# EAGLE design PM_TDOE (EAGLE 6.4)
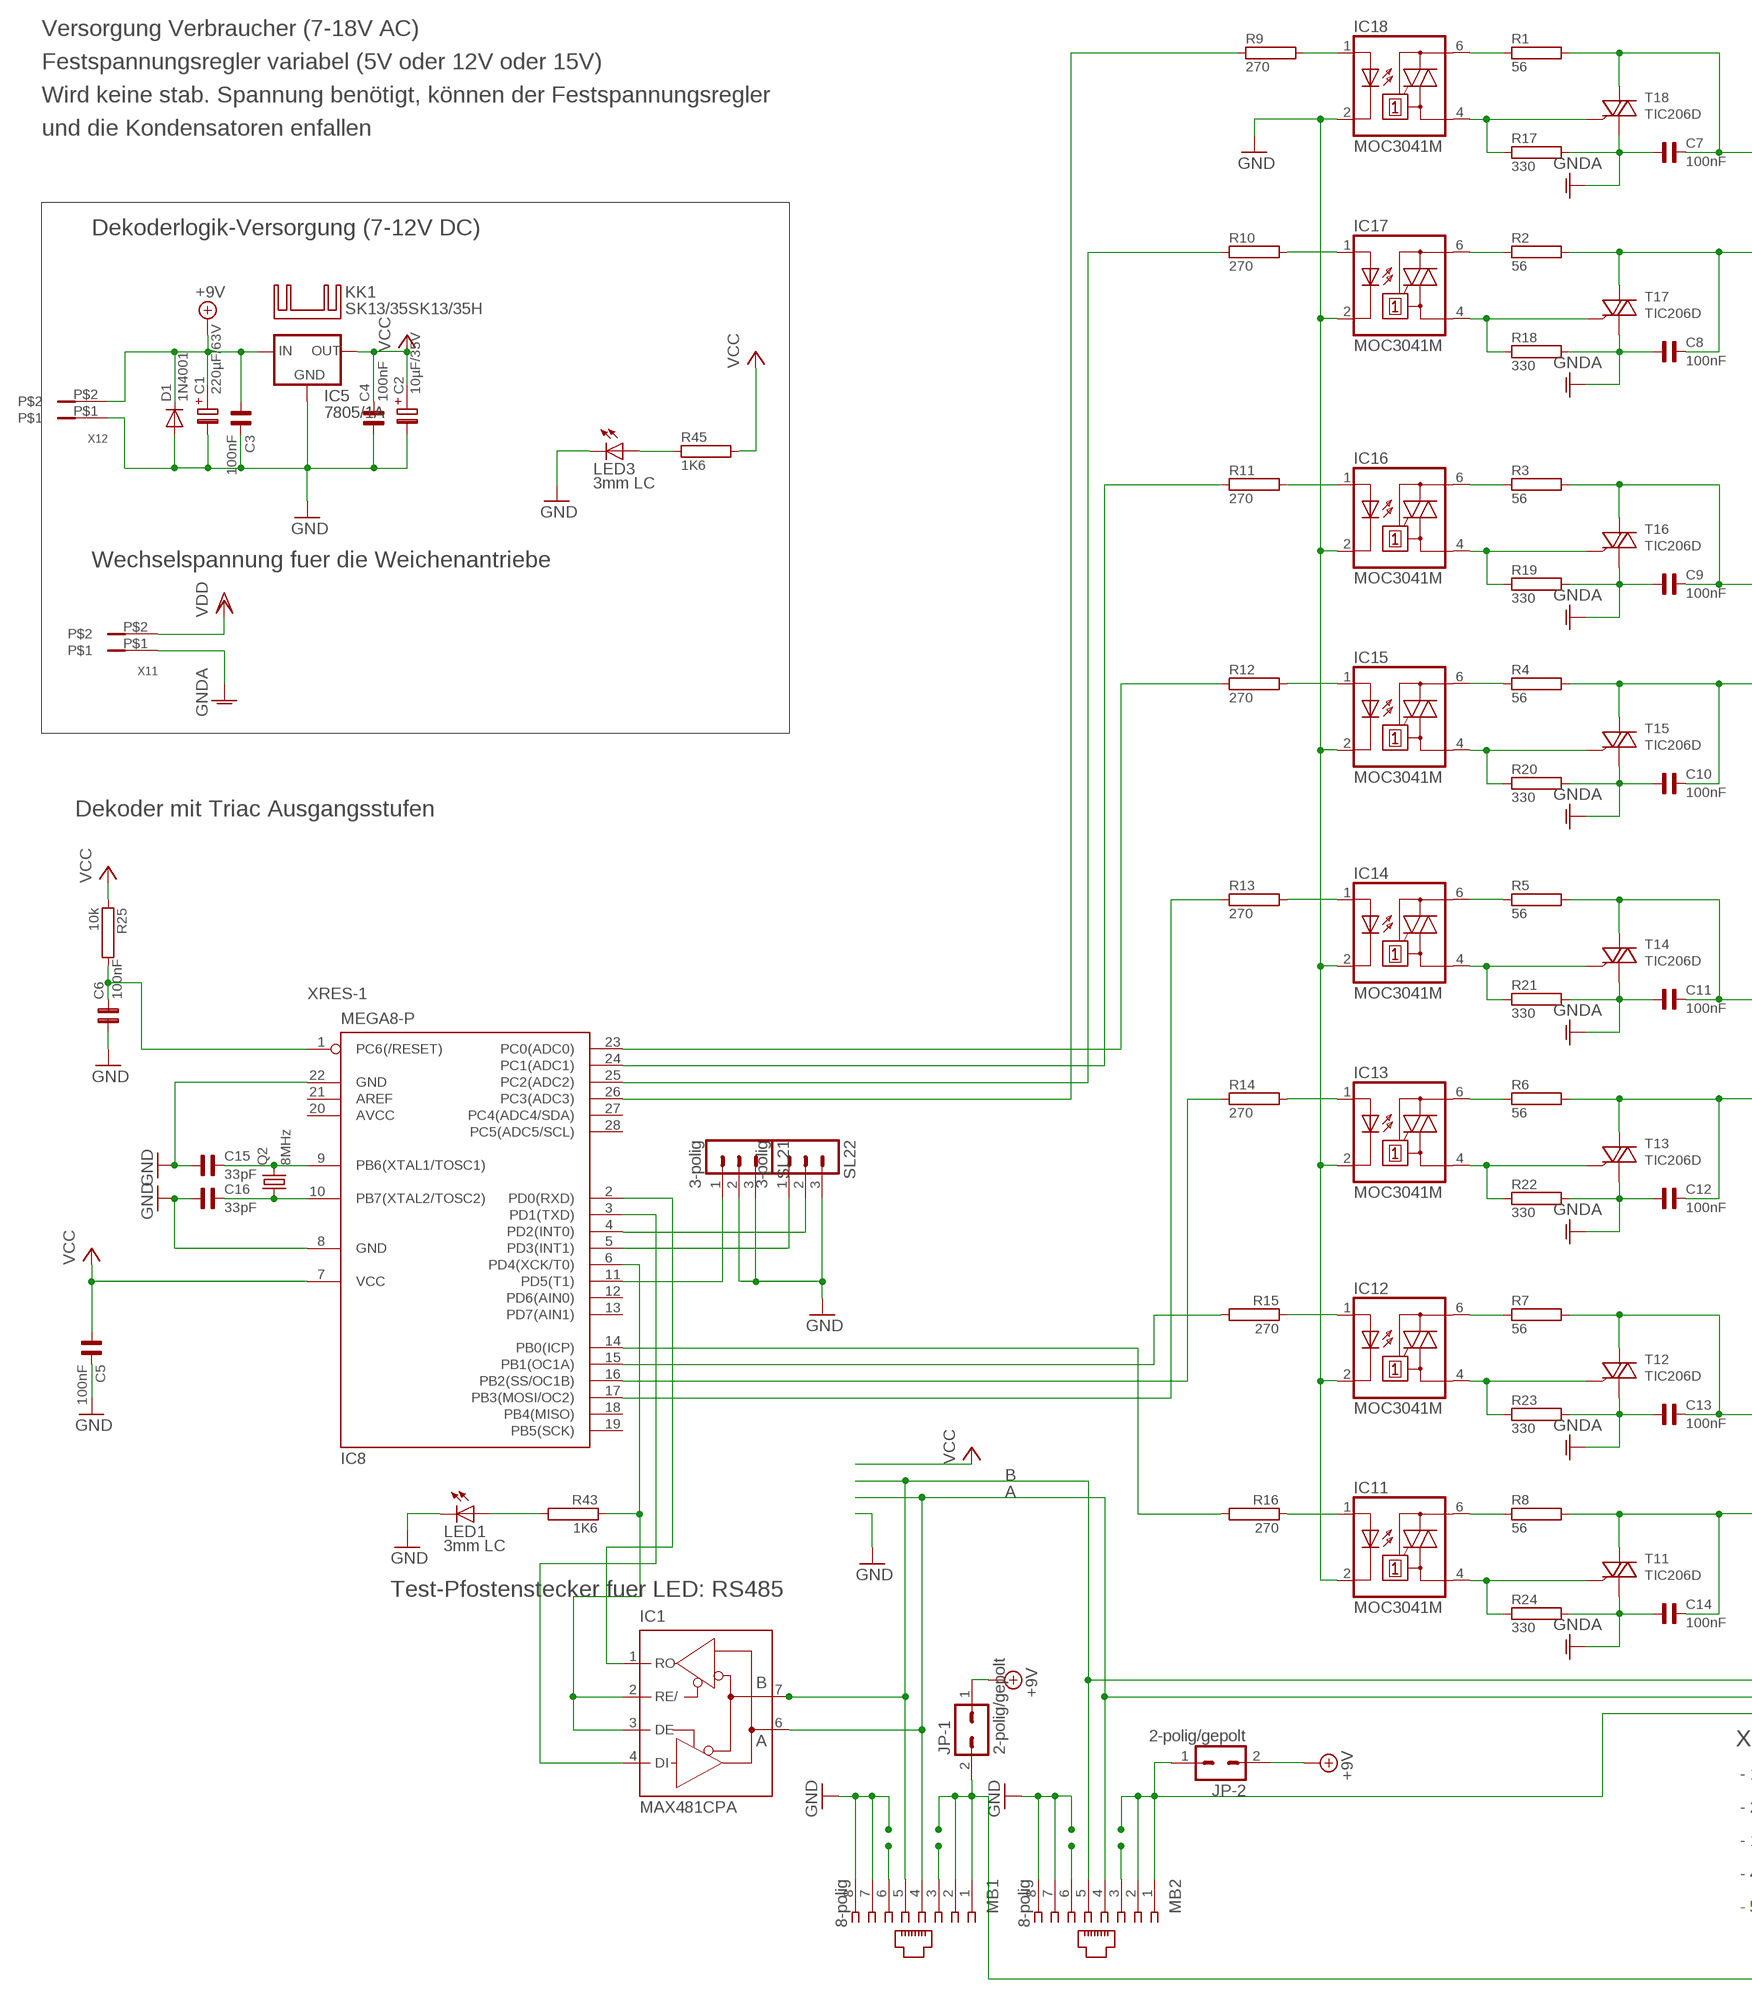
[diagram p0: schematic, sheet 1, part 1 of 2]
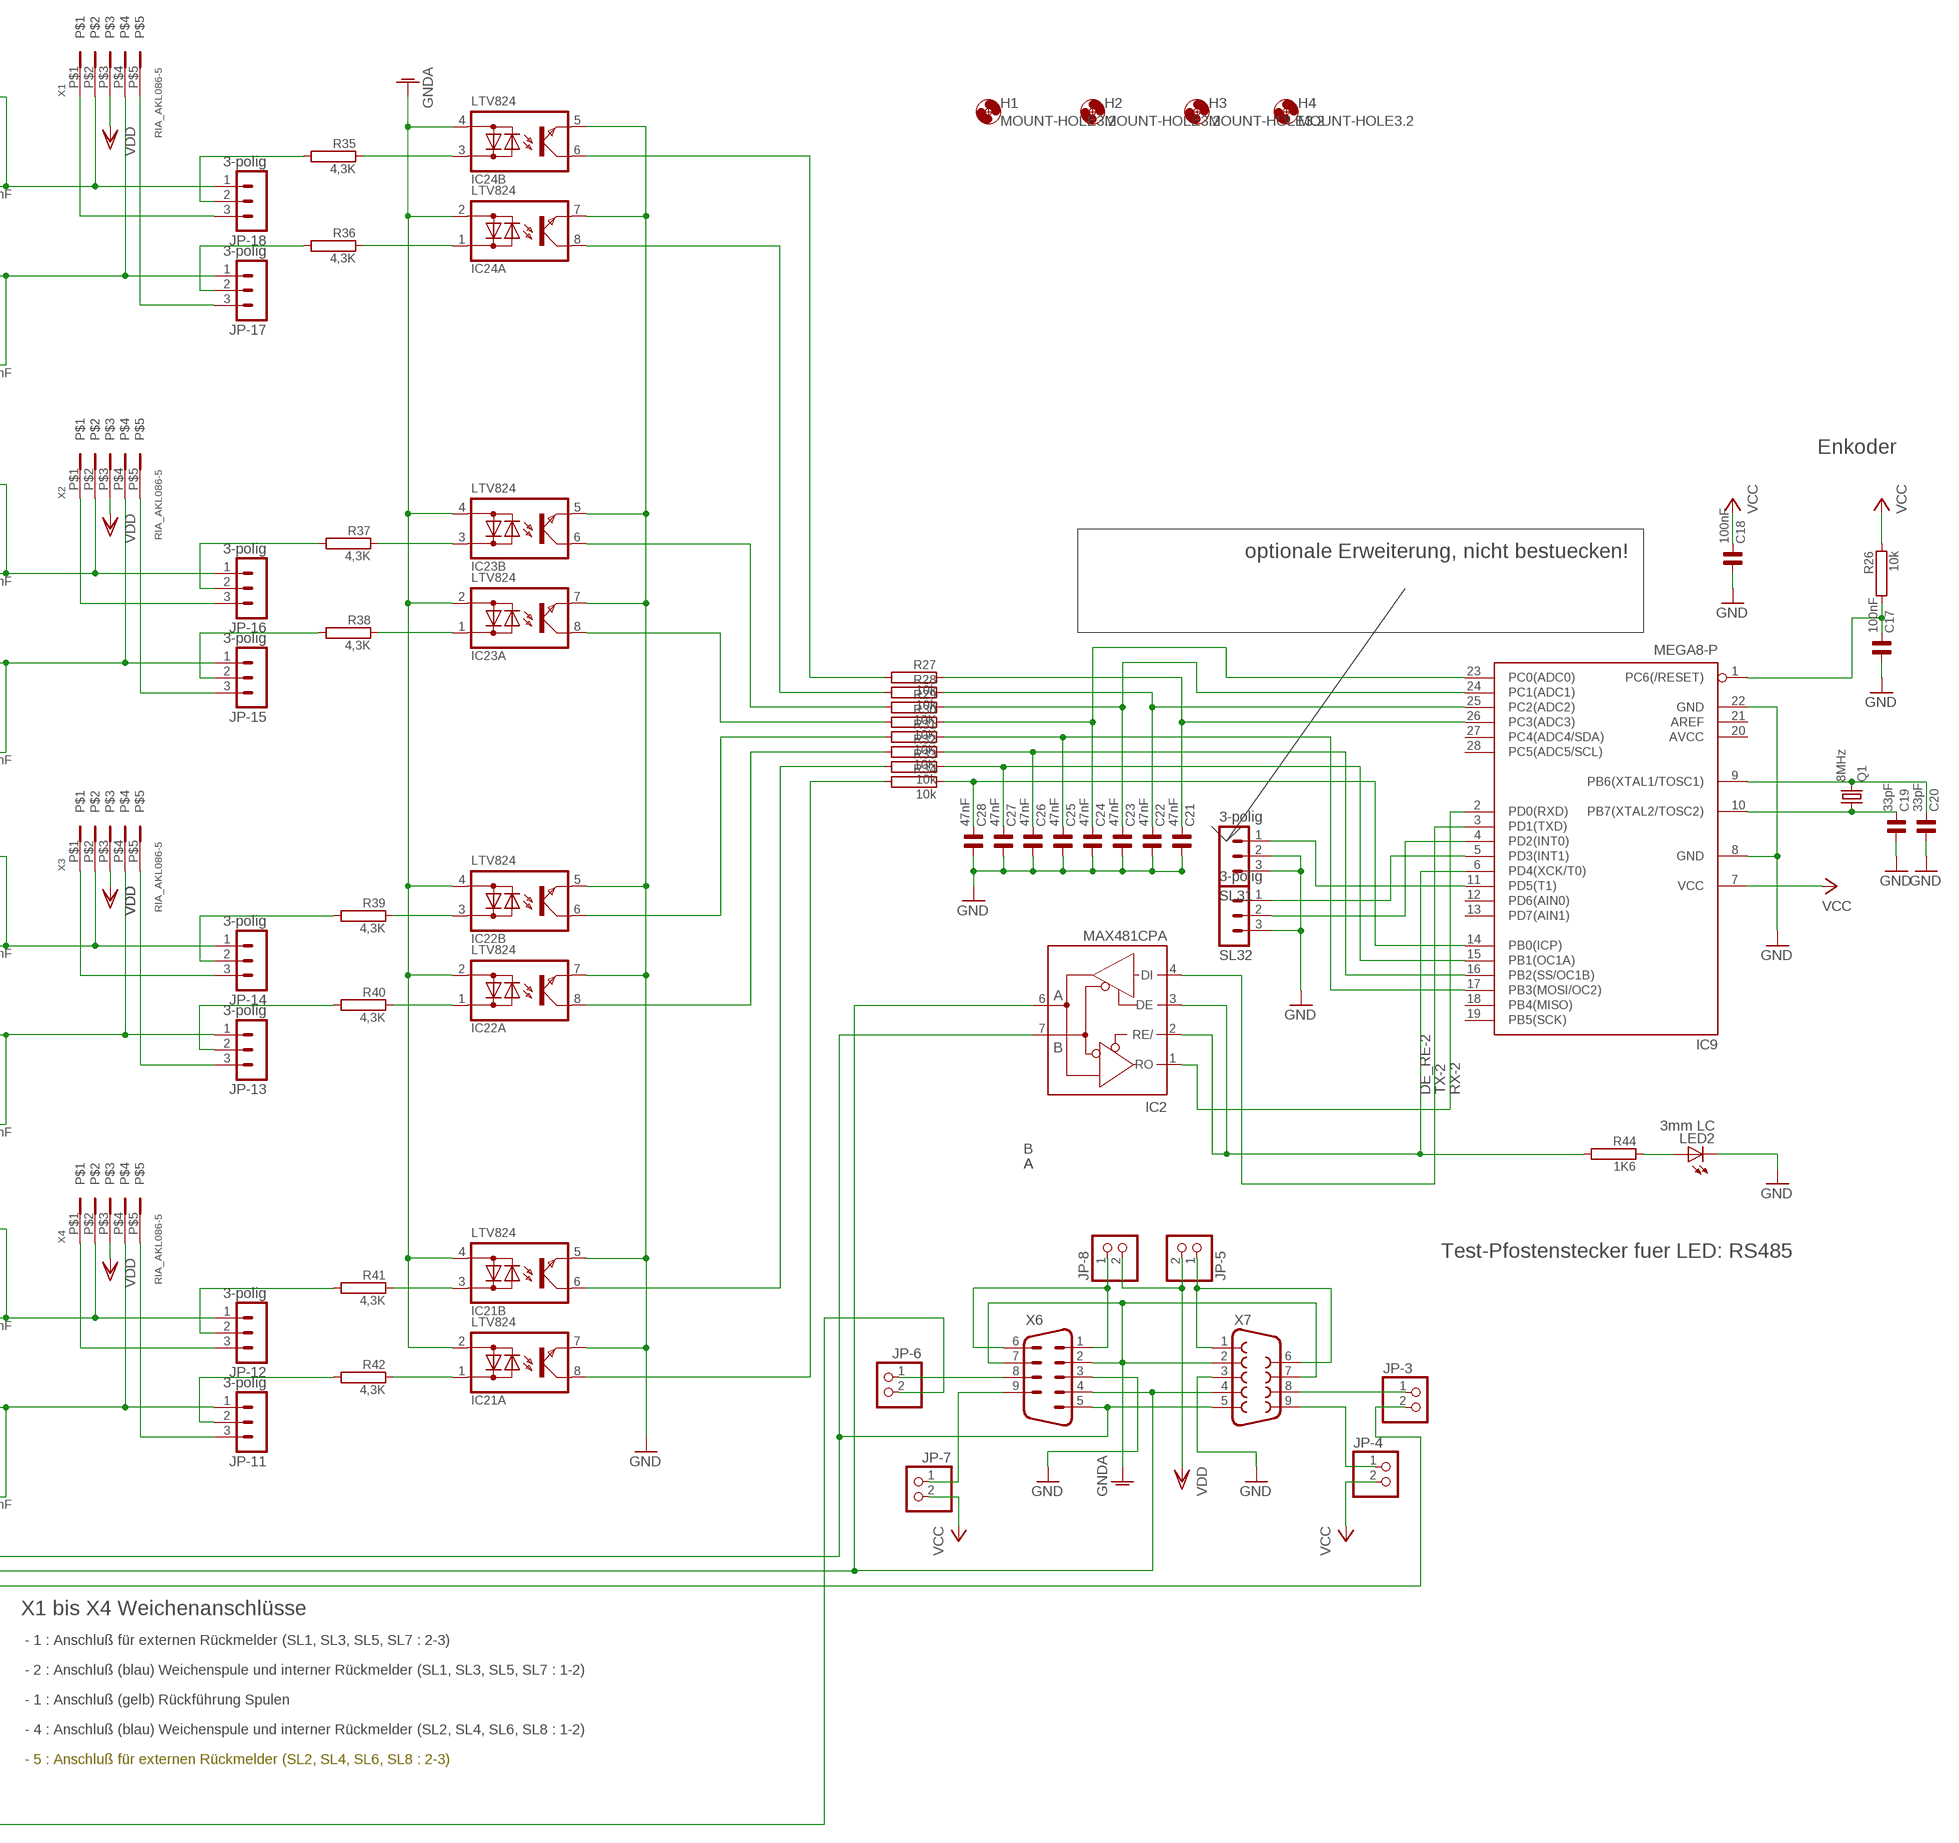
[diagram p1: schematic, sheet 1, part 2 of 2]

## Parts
C1  220µF/63V  E5-10,5  [E5-10,5]
C2  10µF/35V  E2,5-5  [E2,5-5]
C3  100nF  C1206  [1206]
C4  100nF  C1206  [1206]
C5  100nF  C1206  [1206]
C6  100nF  C1206  [1206]
C7  100nF  C1206  [1206]
C8  100nF  C1206  [1206]
C9  100nF  C1206  [1206]
C10  100nF  C1206  [1206]
C11  100nF  C1206  [1206]
C12  100nF  C1206  [1206]
C13  100nF  C1206  [1206]
C14  100nF  C1206  [1206]
C15  33pF  C1206  [1206]
C16  33pF  C1206  [1206]
C17  100nF  C1206  [1206]
C18  100nF  C1206  [1206]
C19  33pF  C1206  [1206]
C20  33pF  C1206  [1206]
C21  47nF  C1206  [1206]
C22  47nF  C1206  [1206]
C23  47nF  C1206  [1206]
C24  47nF  C1206  [1206]
C25  47nF  C1206  [1206]
C26  47nF  C1206  [1206]
C27  47nF  C1206  [1206]
C28  47nF  C1206  [1206]
D1  1N4001  BYM100_1  [SOD-87]
H1  MOUNT-HOLE3.2  [3,2]
H2  MOUNT-HOLE3.2  [3,2]
H3  MOUNT-HOLE3.2  [3,2]
H4  MOUNT-HOLE3.2  [3,2]
IC1  MAX481CPA  [DIL08]
IC2  MAX481CPA  [DIL08]
IC5  7805/1A  78XXS  [78XXS]
IC8  MEGA8-P  [DIL28-3]
IC9  MEGA8-P  [DIL28-3]
IC11  MOC3041M  [DIL06]
IC12  MOC3041M  [DIL06]
IC13  MOC3041M  [DIL06]
IC14  MOC3041M  [DIL06]
IC15  MOC3041M  [DIL06]
IC16  MOC3041M  [DIL06]
IC17  MOC3041M  [DIL06]
IC18  MOC3041M  [DIL06]
IC21  LTV824  [DIL08]
IC22  LTV824  [DIL08]
IC23  LTV824  [DIL08]
IC24  LTV824  [DIL08]
JP-1  2-polig/gepolt  MA01-2  [MA01-2]
JP-2  2-polig/gepolt  MA01-2  [MA01-2]
JP-3  PINHD-1X2  [1X02]
JP-4  PINHD-1X2  [1X02]
JP-5  PINHD-1X2  [1X02]
JP-6  PINHD-1X2  [1X02]
JP-7  PINHD-1X2  [1X02]
JP-8  PINHD-1X2  [1X02]
JP-11  3-polig  MA03-1  [MA03-1]
JP-12  3-polig  MA03-1  [MA03-1]
JP-13  3-polig  MA03-1  [MA03-1]
JP-14  3-polig  MA03-1  [MA03-1]
JP-15  3-polig  MA03-1  [MA03-1]
JP-16  3-polig  MA03-1  [MA03-1]
JP-17  3-polig  MA03-1  [MA03-1]
JP-18  3-polig  MA03-1  [MA03-1]
KK1  SK13/35SK13/35H  [SK13/35H]
LED1  3mm LC  LED3MM  [LED3MM]
LED2  3mm LC  LED3MM  [LED3MM]
LED3  3mm LC  LED3MM  [LED3MM]
MB1  8-polig  555166-1  [555166-1]
MB2  8-polig  555166-1  [555166-1]
Q1  8MHz  HC49/S  [HC49/S]
Q2  8MHz  HC49/S  [HC49/S]
R1  56  R1206  [1206]
R2  56  R1206  [1206]
R3  56  R1206  [1206]
R4  56  R1206  [1206]
R5  56  R1206  [1206]
R6  56  R1206  [1206]
R7  56  R1206  [1206]
R8  56  R1206  [1206]
R9  270  R1206  [1206]
R10  270  R1206  [1206]
R11  270  R1206  [1206]
R12  270  R1206  [1206]
R13  270  R1206  [1206]
R14  270  R1206  [1206]
R15  270  R1206  [1206]
R16  270  R1206  [1206]
R17  330  R1206  [1206]
R18  330  R1206  [1206]
R19  330  R1206  [1206]
R20  330  R1206  [1206]
R21  330  R1206  [1206]
R22  330  R1206  [1206]
R23  330  R1206  [1206]
R24  330  R1206  [1206]
R25  10k  R1206  [1206]
R26  10k  R1206  [1206]
R27  10k  R1206  [1206]
R28  10k  R1206  [1206]
R29  10K  R1206  [1206]
R30  10K  R1206  [1206]
R31  10K  R1206  [1206]
R32  10K  R1206  [1206]
R33  10k  R1206  [1206]
R34  10k  R1206  [1206]
R35  4,3K  R1206  [1206]
R36  4,3K  R1206  [1206]
R37  4,3K  R1206  [1206]
R38  4,3K  R1206  [1206]
R39  4,3K  R1206  [1206]
R40  4,3K  R1206  [1206]
R41  4,3K  R1206  [1206]
R42  4,3K  R1206  [1206]
R43  1K6  R1206  [1206]
R44  1K6  R1206  [1206]
R45  1K6  R1206  [1206]
SL21  3-polig  MA03-1  [MA03-1]
SL22  3-polig  MA03-1  [MA03-1]
SL31  3-polig  MA03-1  [MA03-1]
SL32  3-polig  MA03-1  [MA03-1]
T11  TIC206D  [TO220DS]
T12  TIC206D  [TO220DS]
T13  TIC206D  [TO220DS]
T14  TIC206D  [TO220DS]
T15  TIC206D  [TO220DS]
T16  TIC206D  [TO220DS]
T17  TIC206D  [TO220DS]
T18  TIC206D  [TO220DS]
X1  RIA_AKL086-5  RIA_AKL086-5RIA_AKL086-5  [RIA_AKL086-5]
X2  RIA_AKL086-5  RIA_AKL086-5RIA_AKL086-5  [RIA_AKL086-5]
X3  RIA_AKL086-5  RIA_AKL086-5RIA_AKL086-5  [RIA_AKL086-5]
X4  RIA_AKL086-5  RIA_AKL086-5RIA_AKL086-5  [RIA_AKL086-5]
X6  M09HP  [M09HP]
X7  F09HP  [F09HP]
X11  RIA_AKL086-2  [RIA_AKL086-2]
X12  RIA_AKL086-2  [RIA_AKL086-2]

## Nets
3A: IC8.23(PC0(ADC0)) R12.1
+9V: C1.+ C3.1 D1.2(K) IC5.IN JP-1.1 JP-2.2 X12.P$2
A: IC1.6(A) IC2.6(A) MB1.4 MB2.4 X6.4 X7.4
B: IC1.7(B) IC2.7(B) MB1.5 MB2.5 X6.5 X7.5
DE_RE-1: IC1.2(RE/) IC1.3(DE) IC8.6(PD4(XCK/T0)) R43.1
DE_RE-2: IC2.2(RE/) IC2.3(DE) IC9.6(PD4(XCK/T0)) R44.2
GND: C1.- C2.- C3.2 C4.1 C5.2 C6.1 C15.1 C16.1 C17.1 C18.1 C19.1 C20.1 C21.1 C22.1 C23.1 C24.1 C25.1 C26.1 C27.1 C28.1 D1.1(A) IC5.GND IC8.8(GND) IC8.22(GND) IC9.8(GND) IC11.2(C) IC12.2(C) IC13.2(C) IC14.2(C) IC15.2(C) IC16.2(C) IC17.2(C) IC18.2(C) IC21.5(B:E) IC21.7(A:E) IC22.5(B:E) IC22.7(A:E) IC23.5(B:E) IC23.7(A:E) IC24.5(B:E) IC24.7(A:E) LED1.K(C) LED2.K(C) LED3.K(C) MB1.7 MB1.8 MB2.7 MB2.8 SL21.2 SL21.3 SL22.3 SL31.2 SL31.3 SL32.3 X6.3 X7.3 X12.P$1
GNDA: C7.1 C8.1 C9.1 C10.1 C11.1 C12.1 C13.1 C14.1 IC21.2(A:AK2) IC21.4(B:AK2) IC22.2(A:AK2) IC22.4(B:AK2) IC23.2(A:AK2) IC23.4(B:AK2) IC24.2(A:AK2) IC24.4(B:AK2) R17.2 R18.2 R19.2 R20.2 R21.2 R22.2 R23.2 R24.2 T11.A1 T12.A1 T13.A1 T14.A1 T15.A1 T16.A1 T17.A1 T18.A1 X6.2 X6.7 X7.2 X7.7 X11.P$1
MISO_IF1: IC8.25(PC2(ADC2)) R10.1
MISO_IF2: C22.2 IC9.25(PC2(ADC2)) R28.1
MOSI_IF1: IC8.24(PC1(ADC1)) R11.1
MOSI_IF2: C23.2 IC9.24(PC1(ADC1)) R29.1
N$1: C20.2 IC9.9(PB6(XTAL1/TOSC1)) Q1.2
N$2: C19.2 IC9.10(PB7(XTAL2/TOSC2)) Q1.1
N$3: JP-18.2 R35.2
N$4: IC18.4(A1) R17.1 T18.G
N$5: IC8.11(PD5(T1)) SL21.1
N$6: JP-17.2 R36.2
N$7: IC18.1(A) R9.2
N$8: IC18.6(A2) R1.1
N$9: IC17.1(A) R10.2
N$10: JP-16.2 R37.2
N$11: IC17.6(A2) R2.1
N$12: IC16.1(A) R11.2
N$14: C16.2 IC8.10(PB7(XTAL2/TOSC2)) Q2.1
N$15: IC16.6(A2) R3.1
N$16: IC15.6(A2) R4.1
N$17: IC15.1(A) R12.2
N$18: LED2.A R44.1
N$19: IC14.6(A2) R5.1
N$20: IC14.1(A) R13.2
N$21: IC13.1(A) R14.2
N$22: IC12.1(A) R15.1
N$23: IC13.6(A2) R6.1
N$24: IC12.6(A2) R7.1
N$25: IC11.6(A2) R8.1
N$26: MB2.3
N$27: MB1.6
N$28: MB1.3
N$29: MB2.6
N$30: IC11.1(A) R16.1
N$31: JP-7.1 X6.9
N$32: IC11.4(A1) R24.1 T11.G
N$33: IC12.4(A1) R23.1 T12.G
N$34: IC13.4(A1) R22.1 T13.G
N$35: C14.2 JP-11.1 R8.2 T11.A2 X4.P$4
N$36: C7.2 JP-18.1 R1.2 T18.A2 X1.P$2
N$37: C13.2 JP-12.1 R7.2 T12.A2 X4.P$2
N$38: C9.2 JP-16.1 R3.2 T16.A2 X2.P$2
N$39: C12.2 JP-13.1 R6.2 T13.A2 X3.P$4
N$40: C8.2 JP-17.1 R2.2 T17.A2 X1.P$4
N$41: IC24.6(B:C) R27.2
N$42: IC24.8(A:C) R28.2
N$43: C11.2 JP-14.1 R5.2 T14.A2 X3.P$2
N$44: IC14.4(A1) R21.1 T14.G
N$45: IC23.6(B:C) R29.2
N$46: IC15.4(A1) R20.1 T15.G
N$47: IC23.8(A:C) R30.2
N$48: IC22.6(B:C) R31.2
N$49: IC22.8(A:C) R32.2
N$50: C10.2 JP-15.1 R4.2 T15.A2 X2.P$4
N$51: IC21.6(B:C) R33.2
N$52: IC17.4(A1) R18.1 T17.G
N$53: IC16.4(A1) R19.1 T16.G
N$54: IC21.8(A:C) R34.2
N$55: IC9.11(PD5(T1)) SL31.1
N$56: IC9.5(PD3(INT1)) SL32.1
N$57: IC9.4(PD2(INT0)) SL32.2
N$58: JP-18.3 X1.P$1
N$59: JP-17.3 X1.P$5
N$60: LED1.A R43.2
N$61: LED3.A R45.1
N$62: JP-1.2 JP-6.2 MB1.1 MB1.2
N$63: JP-15.2 R38.2
N$64: JP-2.1 JP-3.2 MB2.1 MB2.2
N$65: IC22.1(A:AK1) R40.1
N$66: IC21.1(A:AK1) R42.1
N$67: IC21.3(B:AK1) R41.1
N$68: IC24.3(B:AK1) R35.1
N$69: IC24.1(A:AK1) R36.1
N$70: IC23.3(B:AK1) R37.1
N$71: IC23.1(A:AK1) R38.1
N$72: IC22.3(B:AK1) R39.1
N$73: JP-4.1 X7.9
N$74: JP-16.3 X2.P$1
N$75: JP-15.3 X2.P$5
N$76: JP-12.3 X4.P$1
N$77: JP-11.3 X4.P$5
N$78: JP-5.1 X7.1 X7.6
N$79: JP-12.2 R41.2
N$80: JP-8.1 X6.1 X6.6
N$81: JP-6.1 X6.8
N$82: JP-14.3 X3.P$1
N$83: JP-13.3 X3.P$5
N$84: JP-14.2 R39.2
N$85: JP-13.2 R40.2
N$86: JP-11.2 R42.2
N$87: JP-3.1 X7.8
N$88: C15.2 IC8.9(PB6(XTAL1/TOSC1)) Q2.2
PB0-1: IC8.14(PB0(ICP)) R16.2
PB0-2: C28.2 IC9.14(PB0(ICP)) R34.1
PB1-1: IC8.15(PB1(OC1A)) R15.2
PB1-2: C27.2 IC9.15(PB1(OC1A)) R33.1
PB2-1: IC8.16(PB2(SS/OC1B)) R14.1
PB2-2: C26.2 IC9.16(PB2(SS/OC1B)) R32.1
PB3-1: IC8.17(PB3(MOSI/OC2)) R13.1
PB3-2: C25.2 IC9.17(PB3(MOSI/OC2)) R31.1
PB4: C24.2 IC9.23(PC0(ADC0)) R30.1
PRG-BUT: IC8.4(PD2(INT0)) SL22.2
RX-2: IC2.1(RO) IC9.2(PD0(RXD))
RXD-1: IC1.1(RO) IC8.2(PD0(RXD))
SCK_IF1: IC8.26(PC3(ADC3)) R9.1
SCK_IF2: C21.2 IC9.26(PC3(ADC3)) R27.1
STATUS: IC8.5(PD3(INT1)) SL22.1
TX-2: IC2.4(DI) IC9.3(PD1(TXD))
TXD-1: IC1.4(DI) IC8.3(PD1(TXD))
VCC: C2.+ C4.2 C5.1 C18.2 IC5.OUT IC8.7(VCC) JP-4.2 JP-7.2 R25.1 R26.1 R45.2
VDD: JP-5.2 JP-8.2 X1.P$3 X2.P$3 X3.P$3 X4.P$3 X11.P$2
XRES-1: C6.2 IC8.1(PC6(/RESET)) R25.2
XRES-2: C17.2 IC9.1(PC6(/RESET)) R26.2
Unconnected: IC8.12(PD6(AIN0)) IC8.13(PD7(AIN1)) IC8.18(PB4(MISO)) IC8.19(PB5(SCK)) IC8.21(AREF) IC8.27(PC4(ADC4/SDA)) IC8.28(PC5(ADC5/SCL)) IC9.12(PD6(AIN0)) IC9.13(PD7(AIN1)) IC9.18(PB4(MISO)) IC9.19(PB5(SCK)) IC9.21(AREF) IC9.27(PC4(ADC4/SDA)) IC9.28(PC5(ADC5/SCL))

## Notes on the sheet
- Versorgung Verbraucher (7-18V AC)
- Festspannungsregler variabel (5V oder 12V oder 15V)
- Wird keine stab. Spannung benötigt, können der Festspannungsregler
- und die Kondensatoren enfallen
- Dekoderlogik-Versorgung (7-12V DC)
- Enkoder
- Wechselspannung fuer die Weichenantriebe | optionale Erweiterung, nicht bestuecken!
- Dekoder mit Triac Ausgangsstufen
- Test-Pfostenstecker fuer LED: RS485
- Test-Pfostenstecker fuer LED: RS485
- X1 bis X4 Weichenanschlüsse
- - 1 : Anschluß für externen Rückmelder (SL1, SL3, SL5, SL7 : 2-3)
- - 2 : Anschluß (blau) Weichenspule und interner Rückmelder (SL1, SL3, SL5, SL7 : 1-2)
- - 1 : Anschluß (gelb) Rückführung Spulen
- - 4 : Anschluß (blau) Weichenspule und interner Rückmelder (SL2, SL4, SL6, SL8 : 1-2)
- - 5 : Anschluß für externen Rückmelder (SL2, SL4, SL6, SL8 : 2-3)

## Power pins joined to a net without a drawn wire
AVCC: IC8.20(AVCC) IC9.20(AVCC)
GND: IC1.5(GND) IC2.5(GND) IC9.22(GND)
VCC: IC1.8(VCC) IC2.8(VCC) IC9.7(VCC)

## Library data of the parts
C1 = POLCAP:E5-10,5
C2 = POLCAP:E2,5-5
C3-C28 = SMD:C1206
D1 = SMD:BYM100_1
H1-H4 = holes:MOUNT-HOLE: MOUNTING HOLE with drill center marker
IC1 IC2 = maxim:MAX481CPA: RS485 TRANSEIVER; MPN: MAX481CPA+; OC_FARNELL: unknown; OC_NEWARK: 99K3445
IC5 = V-REG:78XXS: VOLTAGE REGULATOR
IC8 IC9 = atmel:MEGA8-P: MICROCONTROLLER 8 Kbytes FLASH, 1 kbytes SRAM, 512 bytes EEPROM, USART, 4-channel 10 bit ADC, 2-channel 8 bit ADC Pin compatible with Atmega48, ATMega88, ATMega168 Source: avr.lbr; OC_FARNELL: unknown; OC_NEWARK: unknown
IC11-IC18 = optocoupler:MOC30*: 6-Pin DIP Zero-Cross Optoisolators Triac Driver Output (250/400 Volt Peak) Source: http://www.fairchildsemi.com/ds/MO/MOC3043-M.pdf; MF: FAIRCHILD SEMICONDUCTOR; MPN: MOC3041M; OC_FARNELL: 1086677; OC_NEWARK: 78K6090
IC21-IC24 = LTV824:LTV824
JP-1 JP-2 = CON-LSTB:MA01-2
JP-3-JP-8 = pinhead:PINHD-1X2: PIN HEADER
JP-11-JP-18 SL21 SL22 SL31 SL32 = CON-LSTB@2:MA03-1
KK1 = heatsink:SK13/35: HEATSINK
LED1-LED3 = led:LED: LED
MB1 MB2 = AMP-J:555166-1
Q1 Q2 = QUARTZ:HC49/S
R1-R45 = SMD:R1206
T11-T18 = MoBaSbS:TIC206D
X1-X4 = con-ria_AKL086:RIA_AKL086-5: RIACON AKL086-5
X6 = con-subd:M09: SUB-D; OC_FARNELL: unknown; OC_NEWARK: unknown
X7 = con-subd:F09: SUB-D; OC_FARNELL: unknown; OC_NEWARK: unknown
X11 X12 = con-ria_AKL086:RIA_AKL086-2: RIACON AKL086-2

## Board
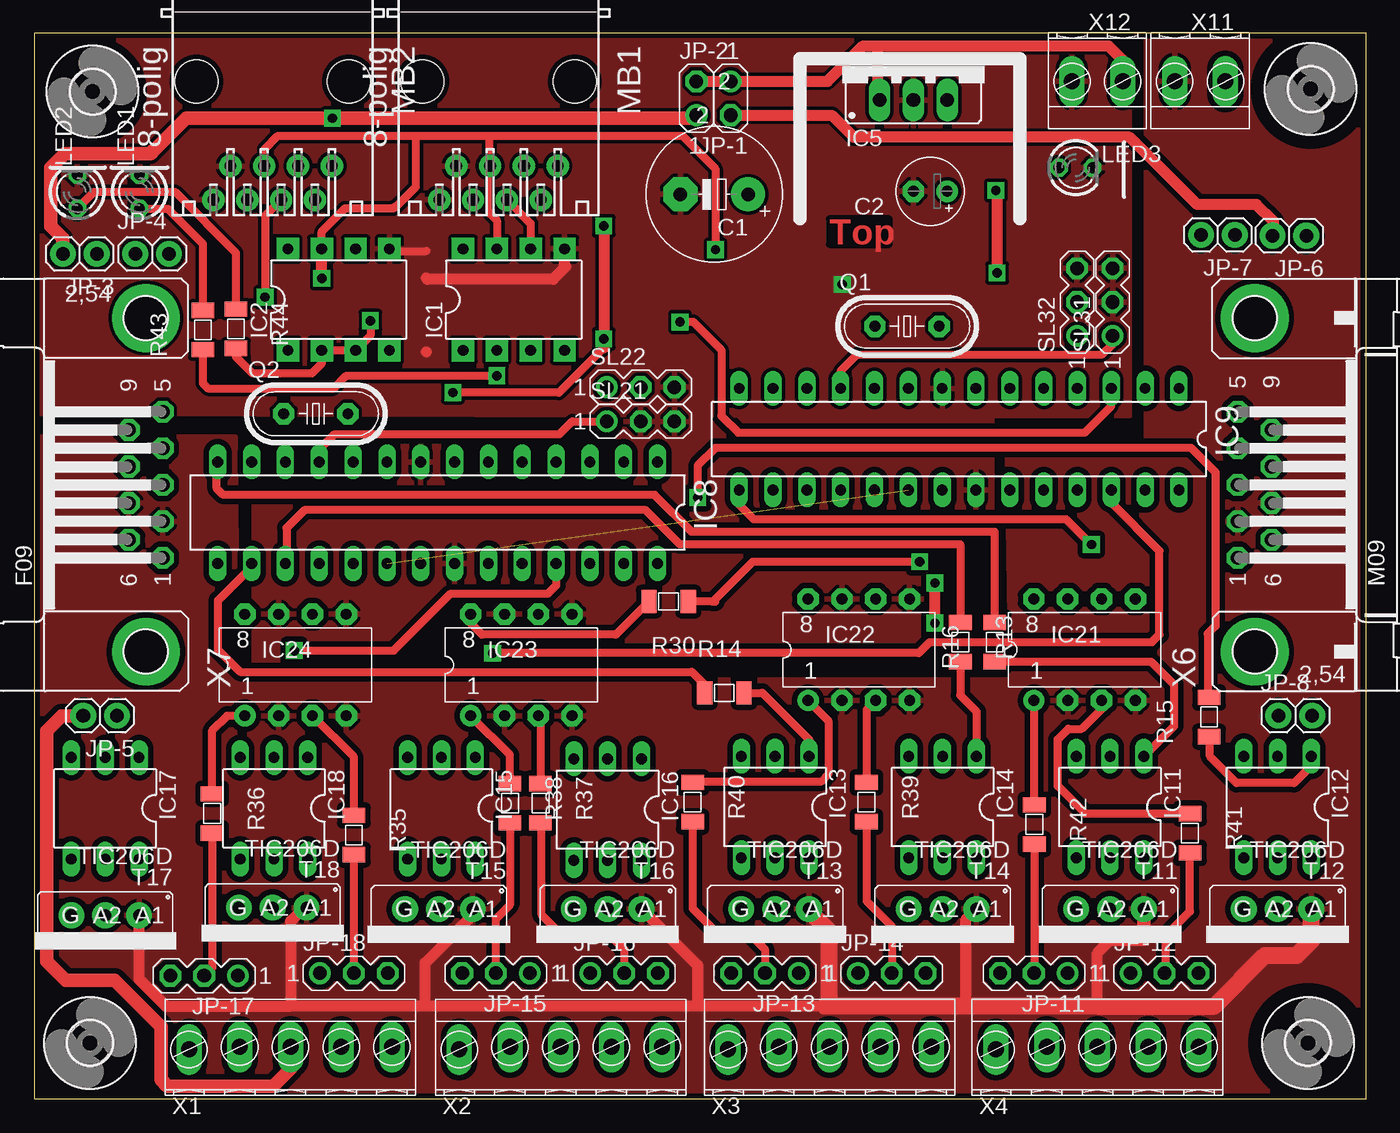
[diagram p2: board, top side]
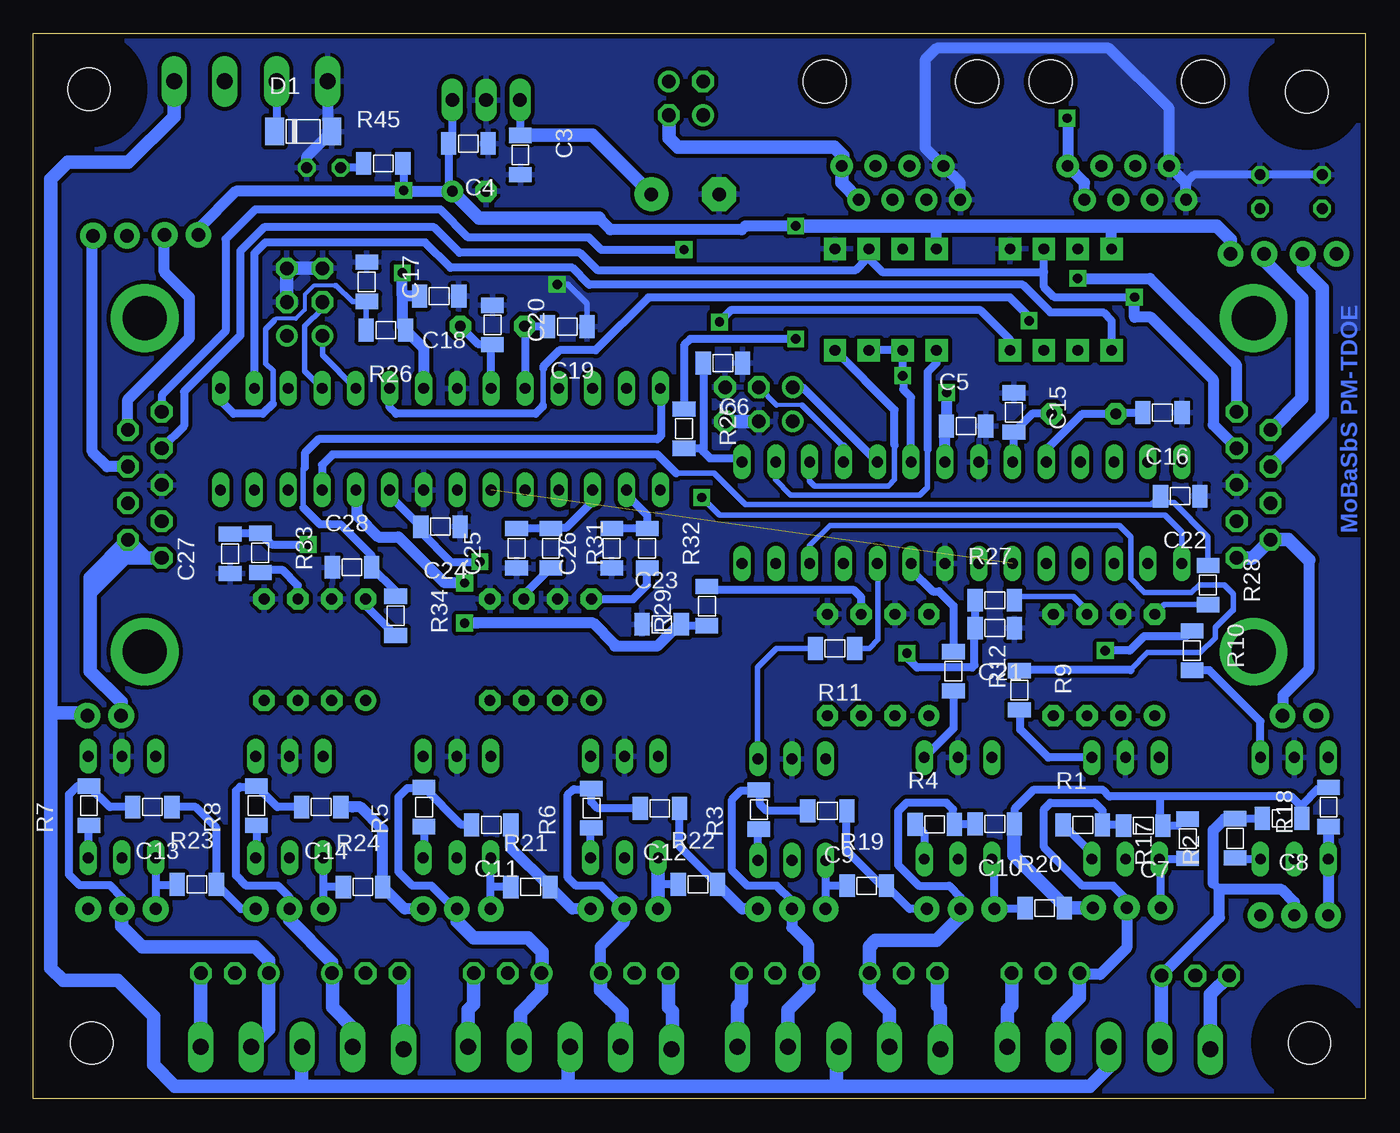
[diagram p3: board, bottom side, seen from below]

Size 100 x 80 mm. Coordinates in mm from the lower left corner, seen from the top.
Outline: 0,0 100,0 100,80 0,80 0,0
Copper layers (1*16): Top 0.035mm / dielectric 1.5mm / Bottom 0.035mm
Design rules "default *": minimum track width 10mil, minimum drill 25mil, track to track 10mil, track to pad 10mil, pad to pad 12mil, via to via 12mil, smd to smd 10mil, copper to edge 15mil, drill to drill 8mil, minimum pad ring 10mil, minimum via ring 10mil, stop-mask expansion 4mil, vias tented up to drill 0mil, thermal gap 10mil

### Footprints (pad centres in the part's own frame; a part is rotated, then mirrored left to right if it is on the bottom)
E5-10,5 = drill 1.016 pad 2.54: + -2.54,0 | drill 1.016 pad 2.54 octagon: - 2.54,0
E2,5-5 = drill 0.813 pad 1.6: + -1.27,0 | drill 0.813 pad 1.6 octagon: - 1.27,0
1206 = smd 1.143 x 1.702: 1 -1.473,0; 2 1.473,0
SOD-87 = smd 1.397 x 2.057: 1 2.134,-0.051; 2 -2.159,-0.051
3,2 = hole 3.2: 0,0
DIL08 = drill 0.813 pad 1.676 square: 1 -3.81,-3.81; 2 -1.27,-3.81; 3 1.27,-3.81; 4 3.81,-3.81; 5 3.81,3.81; 6 1.27,3.81; 7 -1.27,3.81; 8 -3.81,3.81
78XXS = drill 1.016 long: GND 0,-2.54; IN -2.54,-2.54; OUT 2.54,-2.54
DIL28-3 = drill 0.813 long: 1 -16.51,-3.81; 2 -13.97,-3.81; 3 -11.43,-3.81; 4 -8.89,-3.81; 5 -6.35,-3.81; 6 -3.81,-3.81; 7 -1.27,-3.81; 8 1.27,-3.81; 9 3.81,-3.81; 10 6.35,-3.81; 11 8.89,-3.81; 12 11.43,-3.81; 13 13.97,-3.81; 14 16.51,-3.81; 15 16.51,3.81; 16 13.97,3.81; 17 11.43,3.81; 18 8.89,3.81; 19 6.35,3.81; 20 3.81,3.81; 21 1.27,3.81; 22 -1.27,3.81; 23 -3.81,3.81; 24 -6.35,3.81; 25 -8.89,3.81; 26 -11.43,3.81; 27 -13.97,3.81; 28 -16.51,3.81
DIL06 = drill 0.813 long: 1 -2.54,-3.81; 2 0,-3.81; 3 2.54,-3.81; 4 2.54,3.81; 5 0,3.81; 6 -2.54,3.81
DIL08' = drill 0.813 pad 1.6: 1 -3.81,-3.81 | drill 0.813 pad 1.6 octagon: 2 -1.27,-3.81; 3 1.27,-3.81; 4 3.81,-3.81; 5 3.81,3.81; 6 1.27,3.81; 7 -1.27,3.81; 8 -3.81,3.81
MA01-2 = drill 1.016 pad 1.6: 1 0,-1.27 | drill 1.016 pad 1.6 octagon: 2 0,1.27
1X02 = drill 1.016 pad 1.93: 1 -1.27,0; 2 1.27,0
MA03-1 = drill 1.016 pad 1.6: 1 -2.54,0 | drill 1.016 pad 1.6 octagon: 2 0,0; 3 2.54,0
LED3MM = drill 0.813 octagon: A -1.27,0; K 1.27,0
555166-1 = drill 0.889 pad 1.676: 1 -4.445,5.207; 2 -3.175,7.747; 3 -1.905,5.207; 4 -0.635,7.747; 5 0.635,5.207; 6 1.905,7.747; 7 3.175,5.207; 8 4.445,7.747 | hole 3.251: -5.715,-1.143; 5.715,-1.143
HC49/S = drill 0.813 pad 1.6 octagon: 1 -2.413,0; 2 2.413,0
TO220DS = drill 0.9 pad 1.93: A1 -2.54,-2.54; A2 0,-2.54; G 2.54,-2.54
RIA_AKL086-5 = drill 1.2 long: P$1 0,7.62; P$2 0,3.81; P$3 0,0; P$4 0,-3.81; P$5 0.191,-7.62
M09HP = drill 1.016 octagon: 1 -5.486,1.27; 2 -2.743,1.27; 3 0,1.27; 4 2.743,1.27; 5 5.486,1.27; 6 -4.115,-1.27; 7 -1.372,-1.27; 8 1.372,-1.27; 9 4.115,-1.27 | drill 3.302 pad 5.08: G1 -12.522,0; G2 12.522,0
F09HP = drill 1.016 octagon: 1 -5.486,-1.27; 2 -2.743,-1.27; 3 0,-1.27; 4 2.743,-1.27; 5 5.486,-1.27; 6 -4.115,1.27; 7 -1.372,1.27; 8 1.372,1.27; 9 4.115,1.27 | drill 3.302 pad 5.08: G1 -12.522,0; G2 12.522,0
RIA_AKL086-2 = drill 1.2 long: P$1 0,1.905; P$2 0,-1.905

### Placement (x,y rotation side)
C1  51.05,67.91 180 top
C2  67.28,68.14 180 top
C3  63.44,70.87 270 bottom
C4  67.34,71.72 180 bottom
C5  29.97,50.51 0 bottom
C6  48.23,55.24 180 bottom
C7  16.67,20.51 180 bottom
C8  6.25,21.05 180 bottom
C9  40.39,21.62 180 bottom
C10  27.81,20.64 180 bottom
C11  65.63,20.57 180 bottom
C12  52.96,21.81 180 bottom
C13  91.06,21.91 180 bottom
C14  78.39,21.91 180 bottom
C15  26.38,51.53 270 bottom
C16  15.24,51.53 180 bottom
C17  74.96,61.34 270 bottom
C18  69.53,60.26 180 bottom
C19  59.91,57.98 180 bottom
C20  65.53,58.1 270 bottom
C21  27.81,35.34 180 bottom
C22  13.91,45.24 180 bottom
C23  52.83,35.62 0 bottom
C24  69.44,42.96 180 bottom
C25  63.72,41.34 90 bottom
C26  56.58,41.34 90 bottom
C27  85.22,40.93 90 bottom
C28  76.07,39.91 0 bottom
D1  79.72,72.68 0 bottom
H1  4.19,4.19 0 top
H2  95.63,4.19 0 top
H3  95.82,75.82 0 top
H4  4.38,75.63 0 top
IC1  36,60.01 0 top
IC2  22.86,60.01 0 top
IC5  66.01,77.53 0 top
IC8  30.29,44.01 180 top
IC9  69.44,49.53 180 top
IC11  80.77,21.91 180 top
IC12  93.34,21.91 180 top
IC13  55.63,21.91 180 top
IC14  68.2,21.91 180 top
IC15  30.58,21.81 180 top
IC16  43.05,21.72 180 top
IC17  5.33,21.81 180 top
IC18  18,21.81 180 top
IC21  LTV824  [DIL08']  78.87,33.72 0 top
IC22  LTV824  [DIL08']  61.91,33.72 0 top
IC23  LTV824  [DIL08']  36.58,32.58 0 top
IC24  LTV824  [DIL08']  19.62,32.58 0 top
JP-1  52.29,75.12 180 top
JP-2  49.72,75.12 0 top
JP-3  3.43,63.44 180 top
JP-4  8.86,63.44 0 top
JP-5  4.95,28.77 180 top
JP-6  94.23,64.8 180 top
JP-7  88.87,64.87 180 top
JP-8  94.68,28.77 0 top
JP-11  75.06,9.43 180 top
JP-12  84.87,9.43 0 top
JP-13  54.86,9.43 180 top
JP-14  64.39,9.43 0 top
JP-15  34.67,9.43 180 top
JP-16  44.29,9.43 0 top
JP-17  12.76,9.24 180 top
JP-18  24,9.43 0 top
KK1  66.01,78.58 0 top
LED1  7.91,68.1 90 top
LED2  3.24,68.1 90 top
LED3  78.2,69.91 0 top
MB1  34.86,75.25 180 top
MB2  17.91,75.25 180 top
Q1  65.53,58.01 0 top
Q2  21.15,51.44 0 top
R1  21.21,20.57 0 bottom
R2  9.78,19.56 90 bottom
R3  45.53,21.72 90 bottom
R4  32.32,20.61 0 bottom
R5  70.68,21.91 90 bottom
R6  58.1,21.81 90 bottom
R7  95.82,22 90 bottom
R8  83.25,22 90 bottom
R9  25.97,30.67 270 bottom
R10  13.02,33.66 270 bottom
R11  39.81,33.81 180 bottom
R12  30.92,32.1 270 bottom
R13  69.53,34.29 270 top
R14  51.82,30.48 0 top
R15  88.2,28.67 90 top
R16  72.1,34.29 90 top
R17  13.34,19.53 90 bottom
R18  2.76,21.91 90 bottom
R19  37.43,16 0 bottom
R20  24.07,14.32 0 bottom
R21  62.67,15.91 0 bottom
R22  50.1,16.1 0 bottom
R23  87.73,16.1 0 bottom
R24  75.25,15.91 0 bottom
R25  51.15,50.32 270 bottom
R26  73.53,57.72 180 bottom
R27  27.81,37.43 0 bottom
R28  11.81,38.58 270 bottom
R29  49.43,36.99 90 bottom
R30  47.62,37.34 180 top
R31  61.15,41.34 270 bottom
R32  53.91,41.34 270 bottom
R33  82.96,40.99 270 bottom
R34  72.8,36.26 270 bottom
R35  24,19.81 270 top
R36  13.37,21.43 270 top
R37  38,22.19 270 top
R38  35.72,22.19 270 top
R39  62.48,22.29 270 top
R40  49.43,22.29 270 top
R41  86.77,19.94 270 top
R42  75.09,20.61 270 top
R43  12.67,57.72 90 top
R44  15.14,57.82 270 top
R45  73.72,70.23 0 bottom
SL21  45.53,50.86 0 top
SL22  45.53,53.44 0 top
SL31  80.96,59.82 90 top
SL32  78.3,59.82 90 top
T11  80.77,11.72 180 top
T12  93.34,11.72 180 top
T13  55.63,11.72 180 top
T14  68.2,11.72 180 top
T15  30.38,11.72 180 top
T16  43.05,11.72 180 top
T17  5.33,11.24 180 top
T18  17.91,11.81 180 top
X1  19.24,3.91 270 top
X2  39.53,3.91 270 top
X3  59.72,3.91 270 top
X4  79.82,3.91 270 top
X6  91.63,46.1 90 top
X7  8.38,46.1 90 top
X11  87.53,76.39 90 top
X12  79.82,76.39 90 top

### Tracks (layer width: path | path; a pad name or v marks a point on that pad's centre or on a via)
3A
  Bottom 0.61: IC8.23 34.1,39.72 32.48,38.1 32,38.1 30.92,37.02 R12.1
+9V
  Top 0.813: JP-2.2 JP-1.1 59.56,76.39 62.23,79.06 63.34,79.06 | 63.34,79.06 80.64,79.06 81.72,77.98 X12.P$2 | 63.34,75.12 63.34,79.06
  Top 1.016: IC5.IN 63.34,75.12
  Bottom 0.61: X12.P$2 81.72,72.78 D1.2 | IC5.IN 63.47,72.37 C3.1
  Bottom 1.016: C1.+ 58.02,72.34 C3.1
A  (via drill 0.7)
  Top 0.61: MB1.4 37.27,65.72 IC1.6 | MB2.4 17.34,66.29 v17.34,60.2
  Bottom 0.61: 24.13,62.07 24.13,60.96 23.37,60.2 v17.34,60.2 | 24.13,62.07 IC2.6 | X6.4 88.68,50.53 88.68,53.09 84.45,57.31 84.45,63.66 82.68,65.44 69.91,65.44 68.01,63.53 58.96,63.53 57.66,62.23 38.26,62.23 37.4,63.09 37.27,63.09 | 37.27,63.09 IC1.6 | 37.27,63.09 36.26,62.07 24.13,62.07
  Bottom 0.813: v17.34,60.2 17.34,58.67 16.1,58.67 11.43,54.01 11.43,50.62 X7.4
AVCC  (1 unrouted)
B  (via drill 0.7)
  Top 0.305: 34.23,66.55 MB1.5
  Top 0.61: IC2.7 21.59,65.12 23.34,66.86 26.96,66.86 27.05,66.96 27.15,66.96 28.67,68.48 28.67,72.3 | MB2.5 17.27,71.28 18.29,72.3 28.67,72.3 | 28.67,72.3 34.2,72.3 | 34.2,72.3 48.67,72.3 51.15,69.82 v51.15,63.75 | MB1.5 34.2,70.07 34.2,72.3 | 34.23,66.55 34.23,66.45 34.73,65.94 IC1.7
  Top 0.813: v21.59,61.59 IC2.7
  Bottom 0.61: X6.5 90.36,52.83 85.57,57.63 85.57,64.55 83.34,66.77 69.44,66.77 67.34,64.67 58.29,64.67 57.37,63.75 v51.15,63.75
  Bottom 0.813: X7.5 9.65,55.09 16.16,61.59 v21.59,61.59
DE_RE-1  (via drill 0.7)
  Top 0.61: R43.1 12.67,53.72 13.05,53.34 22.48,53.34 23.43,54.29 v34.73,54.29
  Bottom 0.61: IC8.6 34.1,52.67 34.69,53.26 34.69,54.24 v34.73,54.29 IC1.2 IC1.3
DE_RE-2  (via drill 0.7)
  Top 0.61: R44.2 15.14,55.72 16.38,54.48 20.86,54.48 21.59,55.21 IC2.2 IC2.3 25.24,57.31 v25.24,58.42
  Bottom 0.406: 61.72,54.86 61.72,52.1 61.75,52.07
  Bottom 0.61: IC9.6 73.25,51.91 72.77,51.44 62.29,51.44 61.75,51.98 61.75,52.07 | 61.72,54.86 61.72,54.96 60.48,56.2 57.78,56.2 53.82,60.17 26.67,60.17 25.24,58.74 v25.24,58.42
GND  (via drill 0.7)
  Top 0.61: IC2.5 26.83,63.66 29.43,63.66
  Top 0.813: 29.43,61.63 29.53,61.53 38.96,61.53 39.91,62.48 39.81,62.58 IC1.5 | 29.43,56.1
  Bottom 0.406: v60.67,61.15 59.88,61.15 58.42,59.69 58.42,57.99 C19.1
  Bottom 0.61: LED2.K LED1.K 12.86,69.37 13.46,68.77
  Bottom 0.813: MB1.8 30.42,68.77 MB1.7 33.05,71.41 33.05,78.01 32.19,78.87 19.24,78.87 14.73,74.36 MB2.7 13.46,68.77 MB2.8 | X12.P$1 77.92,73.53 77.63,73.25 77.63,72.66 D1.1 79.47,70.75 LED3.K | C15.1 26.71,53
  Bottom 1.016: 65.87,68.28 C2.- 66.01,68.2 | IC5.GND 66.01,75.91 | SL21.3 SL21.2 | SL31.2 SL31.3 SL32.3 | SL32.3
  pour Bottom (isolate 0.305): 0,79.91 0,0 100.01,0 100.11,80.01 5.71,79.63
  pour Top: 0.32,79.69 82.23,79.53 82.23,51.28 0.32,51.44
  pour Top (isolate 0.406): 16.51,52.39 16.51,32.54 71.91,32.54 71.91,52.55 17.14,52.55
GNDA
  Top 0.406: 29.34,6.95 29.34,7.14 29.53,6.95 | 19.24,6.95 19.14,6.95 | 79.92,7.05 79.82,6.95
  Top 0.813: 29.34,6.95 19.24,6.95 | 49.82,6.95 59.34,6.95 59.72,7.33 | 49.82,6.95 29.53,6.95 | 19.24,6.95 9.91,6.95 7.87,8.98 T17.A1 | T18.A1 20.45,14.54 19.24,13.34 19.24,6.95 | 29.34,7.14 29.34,10.19 33.12,13.97 | T16.A1 49.82,10.03 49.82,6.95 | 58.17,14.13 T13.A1 | T14.A1 69.91,13.43 69.91,6.95 | 79.92,7.05 79.82,7.14 79.82,10.95 80.77,11.91 83.25,11.91 83.31,11.97
  Top 1.016: 83.31,11.97 T11.A1
  Top 1.27: 59.34,6.95 69.91,6.95 79.82,6.95 88.58,6.95 92.39,10.76 94.77,10.76 95.89,11.87 T12.A1 | 59.72,7.33 59.72,12.57 58.17,14.13
  Bottom 0.61: R17.2 13.48,21.15 14.12,20.51 C7.1 15.4,20.71 15.4,22.7 | T15.A1 34.21,14.26 R19.2 36.29,16 38.96,18.67 38.96,21.58 C9.1 | R22.2 51.49,18.95 C12.1 | C14.1 | T11.A1 84.41,14.26 R23.2 86.25,20.34 87.82,21.91 C13.1 | 4.78,21.93 4.78,22.05 3.49,23.34 2.81,23.34 R18.2 | C8.1 4.78,21.93 | C10.1 26.34,21.76 24.92,23.18 19.68,23.18 19.21,22.7 15.4,22.7 | 4.78,21.93 5.56,22.7 15.4,22.7
  Bottom 0.813: T16.A1 46.79,14.26 R22.2 | T13.A1 59.55,14.26 R21.2 64.15,18.86 C11.1 | T14.A1 72.12,14.26 R24.2 73.77,20.24 75.44,21.91 76.04,21.91 C14.1
  Bottom 1.016: 21.83,14.35 T18.A1 22.45,14.35 | 22.45,14.35 26.38,18.29 26.38,20.59 C10.1 | R20.2 22.56,14.35 22.45,14.35
  pour Top (isolate 0.406): 83.5,79.85 83.5,48.1 99.54,48.1 99.54,79.85
  pour Top (isolate 0.406): 0.32,49.69 15.08,49.69 15.24,31.43 73.34,31.43 73.03,50.16 99.54,50.16 99.69,0.32 0.32,0.32
MISO_IF1  (via drill 0.7)
  Top 0.61: v19.53,33.66 26.99,33.66 31.27,37.94 38.58,37.94 39.21,38.58 39.21,40.16 IC8.25
  Bottom 0.406: 13.43,34.72 R10.1
  Bottom 0.61: 13.43,34.72 16.62,34.72 17.68,33.66 v19.53,33.66
MISO_IF2
  Bottom 0.254: 76.2,48.26 76.2,48.39
  Bottom 0.406: 15.53,44.77 15.91,44.77 16.05,44.62 46.53,44.62 48.9,46.99 51.69,46.99 51.72,46.96 | 15.53,44.77 15.38,44.91 C22.2 | 15.53,44.77 14.38,44.77 11.81,42.2 R28.1
  Bottom 0.61: 51.72,46.96 53.15,48.39 76.2,48.39 77.53,48.39 78.33,47.59 IC9.25
MOSI_IF1
  Bottom 0.406: R11.1 37.24,33.81 36.58,34.48 36.58,40.13 IC8.24
MOSI_IF2  (via drill 0.7)
  Top 0.813: v67.63,35.72 v67.63,38.73
  Bottom 0.61: R29.1 51.25,35.52 C23.2 51.53,35.62 | 56.36,33.97 56.36,34.13
  Bottom 0.813: 66.67,35.72 v67.63,35.72 57.94,35.72 56.36,34.13 | IC9.24 75.69,45.72 75.69,43.78 74.11,42.2 72.58,42.2 69.12,38.73 v67.63,38.73 | 51.53,35.62 53.18,33.97 56.36,33.97
N$1
  Bottom 0.61: Q1.2 66.57,56.63 C20.2 65.63,56.53 IC9.9
N$2
  Bottom 0.61: C19.2 63.09,57.98 | 63.09,57.98 Q1.1 | 63.09,57.98 IC9.10 | IC9.10
N$3
  Top 0.61: JP-18.2 R35.2
N$4
  Bottom 0.61: T18.G 15.37,17.91 IC18.4 13.39,18 R17.1
N$5
  Top 0.61: SL21.1 40.39,50.86 39.43,49.91 22.57,49.91 21.34,48.67 21.34,47.88 IC8.11
N$6
  Top 0.61: R36.2 13.37,9.84 JP-17.2
N$7
  Bottom 0.61: IC18.1 23.81,25.62 25.91,27.72 25.91,29.13 R9.2
N$8
  Bottom 0.61: IC18.6 20.54,18.43 R1.1
N$9
  Bottom 0.61: 12.7,32.5 R10.2 11.7,32.18 7.87,28.35 IC17.1
N$10
  Top 0.61: R37.2 38.1,20.62 38.1,13.81 39.43,12.48 43.05,12.48 44.29,11.24 JP-16.2
N$11
  Bottom 0.61: R2.1 9.7,18 IC17.6
N$12
  Bottom 0.406: R11.2 44.2,33.81 45.62,32.38 45.62,25.56 IC16.1
N$14
  Bottom 0.61: IC8.10 23.94,48.74 21.24,51.44 Q2.1 18.64,51.53 C16.2
N$15
  Bottom 0.61: IC16.6 45.59,20.18 R3.1
N$16
  Bottom 0.61: R4.1 33.12,19.93 IC15.6
N$17
  Bottom 0.61: R12.2 30.92,27.81 IC15.1
N$18
  Top 0.61: LED2.A 4.51,68.1 10.57,68.1 15.14,63.53 R44.1
N$19
  Bottom 0.61: R5.1 70.67,18.16 IC14.6
N$20
  Top 0.61: R13.2 69.53,30.29 70.74,29.08 IC14.1
N$21
  Top 0.61: R14.2 54.67,30.48 58.2,26.96 58.2,25.75 IC13.1
N$22
  Top 0.61: IC12.1 95.82,25.65 95.82,24.96 94.58,23.72 90.27,23.72 88.27,25.72 88.27,27.13 R15.1
N$23
  Bottom 0.61: IC13.6 58.17,20.28 R6.1
N$24
  Bottom 0.61: IC12.6 95.82,18.16 R7.1
N$25
  Bottom 0.61: R8.1 83.25,18.16 IC11.6
N$30
  Top 0.61: 83.34,25.75 IC11.1 85.57,27.97 85.57,31.11 83.86,32.82 R16.1
N$31
  Bottom 0.813: X6.9 92.9,52.51 88.27,57.15 88.27,60.17 90.17,62.07 90.17,64.83 JP-7.1
N$32
  Bottom 0.61: IC11.4 78.23,15.91 | 78.23,15.91 T11.G | R24.1 78.23,15.91 | 78.23,15.91
N$33
  Bottom 0.61: IC12.4 90.81,16.03 | 90.81,16.03 T12.G | R23.1 89.26,16.03 90.81,16.03
N$34
  Bottom 0.61: R22.1 52.99,16.1 53.09,16
  Bottom 1.016: T13.G 53.09,16 IC13.4
N$35
  Bottom 0.61: C14.2 81.68,21.91 R8.2 83.29,23.43 84.49,23.43 84.77,23.15 84.77,16.76 84.01,16 81.63,16 80.77,15.14 T11.A2
  Bottom 0.813: 77.53,9.37 JP-11.1
  Bottom 1.016: X4.P$4 76.01,5.33 77.53,6.86 77.53,9.37 | T11.A2 80.77,13.43 77.6,10.26 JP-11.1
N$36
  Bottom 0.61: T18.A2 17.91,14.95 18.95,16 21.24,16 24.13,18.89 24.13,21.75 23.65,22.23 20.32,22.23 19.74,21.64 R1.2 | R1.2 19.84,20.48 | C7.2 18.21,20.57 R1.2
  Bottom 0.813: 23.05,6 X1.P$2 | T18.A2 17.91,11.34 19.91,9.34 21.37,9.34 JP-18.1
  Bottom 1.016: JP-18.1 21.46,7.59 23.05,6
N$37
  Bottom 0.61: C13.2 94.25,21.91 R7.2 | T12.A2 93.34,15.14 94.23,16.03 96.52,16.03 97.31,16.83 97.31,22.86 96.68,23.5 95.84,23.5 R7.2 | 95.87,23.43 R7.2
  Bottom 1.016: T12.A2 93.34,12.95 91.82,11.43 83.34,11.43 82.33,10.41 JP-12.1 82.33,5.21 X4.P$2
N$38
  Bottom 0.61: C9.2 44.96,21.62 45.43,22.1 45.43,23.09 R3.2 45.57,23.15 46.86,23.15 47.53,22.48 47.53,17.14 46.39,16 44.2,16 43.05,14.86 T16.A2
  Bottom 0.813: T16.A2 43.05,12.86 41.81,11.62 41.81,9.49 JP-16.1
  Bottom 1.016: JP-16.1 41.75,8.26 43.34,6.67 X2.P$2
N$39
  Bottom 0.61: C12.2 57.63,21.81 58.1,22.29 R6.2 | R6.2 | T13.A2 57.37,16 59.24,16 59.91,16.67 59.91,22.77 59.44,23.24 58.15,23.24 R6.2
  Bottom 0.813: T13.A2 55.63,13.24 57.44,11.43 57.44,9.46 JP-13.1 | 55.82,4 X3.P$4
  Bottom 1.016: JP-13.1 57.4,8.16 55.82,6.57 55.82,4
N$40
  Bottom 0.61: 10.56,21.03 R2.2 9.76,21.05 C8.2 | 10.95,15.72 11.43,16.19
  Bottom 0.813: T17.A2 5.33,14.76 6.29,15.72 10.95,15.72 10.95,13.62 15.3,9.27 15.34,9.27 JP-17.1 | 11.43,16.19 11.43,20.16 10.56,21.03
  Bottom 1.016: JP-17.1 15.3,4.03 X1.P$4
N$41
  Bottom 0.406: IC24.6 20.89,36.7 21.91,37.72 26.05,37.72 R27.2
N$42
  Bottom 0.406: R28.2 15.09,37.1 IC24.8
N$43
  Bottom 0.61: C11.2 67.87,20.57 R5.2 70.72,23.34 71.91,23.34 72.58,22.67 72.58,17.05 71.53,16 70.1,16 68.36,14.26 T14.A2
  Bottom 0.813: 61.82,9.46 JP-14.1 | 63.44,4 X3.P$2
  Bottom 1.016: T14.A2 68.2,13.34 66.96,12.1 62.87,12.1 61.82,11.05 61.82,9.46 | JP-14.1 61.85,8.06 63.44,6.48 63.44,4
N$44
  Bottom 0.61: T14.G 65.66,15.91 | 65.66,15.91 IC14.4 | R21.1 65.66,15.91
N$45
  Bottom 0.61: IC23.6 37.85,37.66 38.39,38.2 49.17,38.2 R29.2
N$46
  Bottom 0.61: IC15.4 27.84,17.81 T15.G 25.6,14.26 R20.1
N$47
  Top 0.61: IC23.8 32.77,35.72 33.62,34.86 43.67,34.86 R30.2
N$48
  Bottom 0.61: IC22.6 63.18,37.83 R31.2
N$49
  Bottom 0.61: IC22.8 54.96,37.53 53.91,38.58 R32.2
N$50
  Bottom 0.61: T15.A2 30.39,15.14 31.24,16 33.53,16 35.08,17.56 35.08,21.59 34.45,22.23 31.43,22.23 30.96,21.75 30.96,20.71 R4.2 29.32,20.61 C10.2
  Bottom 0.813: 37.24,9.46 JP-15.1 | T15.A2 30.39,13.72 30.96,13.14
  Bottom 1.016: 30.57,13.53 30.96,13.14 32.19,11.91 36.77,11.91 37.24,11.43 37.24,9.46 | JP-15.1 37.21,8.06 35.72,6.57 X2.P$4
N$51
  Bottom 0.61: IC21.6 80.14,38.54 81.28,39.69 82.79,39.69 R33.2
N$52
  Bottom 0.813: R18.1 2.79,20.4 IC17.4 T17.G
N$53
  Bottom 0.61: IC16.4 40.51,16 | 40.51,16 T16.G | R19.1 40.51,16
N$54
  Bottom 0.61: IC21.8 75.06,37.04 R34.2
N$55
  Top 0.61: IC9.11 60.55,54.64 61.78,55.88 80.17,55.88 80.96,56.67 SL31.1
N$56
  Bottom 0.406: SL32.1 78.3,55.85 IC9.5
N$57
  Bottom 0.406: IC9.4 79.63,54.64 79.63,58.01 78.3,59.34 SL32.2
N$58
  Bottom 1.016: JP-18.3 26.54,6.99 26.86,6.67 X1.P$1
N$59
  Bottom 1.016: JP-17.3 11.62,7.84 X1.P$5
N$60
  Top 0.61: LED1.A 10.03,66.83 12.67,64.2 R43.2
N$61
  Bottom 0.61: R45.1 75.51,69.91 LED3.A
  Bottom 1.016: LED3.A 76.82,69.91
N$62
  Top 0.813: JP-1.2 59.88,73.85 61.53,72.2 82.26,72.2 87.31,67.15 91.76,67.15 93.03,65.88 93.03,64.86
  Top 1.016: 93.03,64.86 JP-6.2
  Bottom 1.016: MB1.1 39.31,68.77 MB1.2 | MB1.1 39.31,70.07 | MB1.1 39.34,70.01 | JP-1.2 52.29,72.14 51.59,71.44 39.85,71.44 39.21,70.8 39.21,70.14 MB1.1
N$63
  Top 0.61: JP-15.2 34.67,13.53 35.72,14.57 R38.2
N$64  (via drill 0.7)
  Top 1.016: JP-3.2 2.16,64.61 1.24,65.53 1.24,69.91 2.29,70.96 8.73,70.96 9.02,71.25 9.05,71.25 11.43,73.63 v22.38,73.63 49.5,73.63 JP-2.1
  Bottom 0.813: MB2.2 21.08,68.77 | 21.08,68.77 MB2.1 | 21.08,68.77 21.08,68.8 22.29,70.01 22.29,73.53 v22.38,73.63
N$65
  Top 0.61: IC22.1 59.63,28.38 59.63,24.38 59.05,23.81 49.49,23.81 R40.1
N$66
  Top 0.61: IC21.1 75.06,22.11 R42.1
N$67
  Top 0.61: IC21.3 80.14,29.27 78.64,27.78 77.63,27.78 76.83,26.99 76.83,23.5 78.9,21.43 86.75,21.43 R41.1
N$68
  Top 0.61: R35.1 24,25.65 IC24.3
N$69
  Top 0.61: IC24.1 14.48,28.77 13.34,27.62 13.34,22.94 R36.1
N$70
  Top 0.61: IC23.3 38.01,28.61 R37.1
N$71
  Top 0.61: IC23.1 35.72,25.81 R38.1
N$72
  Top 0.61: IC22.3 62.48,29.21 R39.1
N$73
  Bottom 1.016: X7.9 4.76,52.56 4.76,60.1 7.53,62.87 | 7.53,62.87 | 7.53,62.87 7.53,63.37 JP-4.1
N$74
  Bottom 1.016: JP-16.3 46.83,7.27 47.15,6.95 X2.P$1
N$75
  Bottom 1.016: JP-15.3 32.13,6.99 31.91,6.76 X2.P$5
N$76
  Bottom 0.813: JP-12.3 87.44,9.4
  Bottom 1.016: 87.44,9.4 X4.P$1
N$77
  Bottom 1.016: X4.P$5 72.2,9.11 JP-11.3
N$78
  Bottom 0.813: 4.25,40.45 4.25,32.23 6.19,30.29 6.19,28.8 JP-5.1
  Bottom 1.016: X7.1 8.48,40.62 X7.6 5.79,41.99 4.25,40.45
N$79
  Top 0.61: JP-12.2 84.93,9.49 84.93,12.22 86.77,14.06 R41.2
N$80
  Bottom 1.016: 92.16,41.25 X6.6 95.73,39.16 95.73,32.1 93.41,29.78 JP-8.1 | 92.16,41.25 91.53,40.61 X6.1 93.12,40.61 95.63,38.1 | 92.16,41.25 93.34,41.25 93.53,41.05
N$81
  Bottom 0.813: X6.8 94.46,47.47 95.57,48.58 95.57,64.74 JP-6.1
N$82
  Bottom 1.016: JP-14.3 66.93,7.08 67.34,6.67 X3.P$1
N$83
  Bottom 0.813: 52.01,3.81 X3.P$5
  Bottom 1.016: JP-13.3 52.32,6.89 52.01,6.57 52.01,3.81
N$84
  Top 0.61: JP-14.2 64.39,12.95 62.48,14.86 R39.2
N$85
  Top 0.61: R40.2 49.44,14.29 51.24,12.48 53.63,12.48 54.86,11.24 JP-13.2
N$86
  Top 0.61: R42.2 75.09,9.46 JP-11.2
N$87
  Bottom 1.016: JP-3.1 4.7,62.99 4.67,62.96 4.67,62.29 3.24,60.87 3.24,51.35 X7.8
N$88
  Bottom 0.61: IC8.9 26.38,47.82 C15.2 25.01,51.44 Q2.2
PB0-1
  Top 0.61: 13.78,47.66 IC8.14 13.72,47.75 13.72,45.81 14.19,45.34 46.58,45.34 49.34,42.58 72.1,42.58 R16.2
PB0-2
  Bottom 0.406: 79.63,47.43 79.72,47.34 79.72,44.39
  Bottom 0.61: IC9.14 52.86,53.28 52.86,49.82 53.15,49.53 78.58,49.53 79.63,48.48 79.63,47.43 | 79.72,44.39 78.49,43.15 76.96,43.15 74.61,40.8 74.61,39.92 C28.2 72.8,38.11 R34.1
PB1-1  (via drill 0.7)
  Top 0.61: v49.82,45.15 49.82,47.53 51.15,48.86 86.87,48.86 88.68,47.05 88.68,35.5 88.11,34.92 88.11,30.24 R15.2
  Bottom 0.406: v49.82,45.15 48.48,43.81 15.05,43.81 13.78,42.55 IC8.15
PB1-2  (via drill 0.7)
  Top 0.61: IC9.15 52.93,44.61 54.01,43.53 77.47,43.53 v79.38,41.62
  Bottom 0.61: C27.2 85.15,42.46 R33.1 82.12,41.62 v79.38,41.62
PB2-1
  Top 0.61: IC8.16 16.32,39.94 13.81,37.43 13.81,33.72 15.46,32.07 49.37,32.07 50.32,31.11 50.32,30.5 R14.1
PB2-2
  Bottom 0.61: C26.2 R32.1 53.91,43.81 55.47,45.37 IC9.16
PB3-1
  Top 0.61: R13.1 69.53,41.62 48.48,41.62 45.91,44.2 20.29,44.2 18.95,42.86 18.95,40.29 IC8.17
PB3-2
  Bottom 0.61: 63.15,42.81 C25.2 | IC9.17 58.01,44.86 60.01,42.86 61.1,42.86 R31.1 63.15,42.81 | 63.15,42.81
PB4  (via drill 0.7)
  Top 0.61: 51.15,37.34 50.96,37.34 | 50.96,37.34 R30.1 | v66.48,40.32 53.94,40.32 50.96,37.34
  Bottom 0.61: IC9.23 73.25,45.3 C24.2 70.91,42.58 68.66,40.32 v66.48,40.32
PRG-BUT
  Bottom 0.305: 42.29,52.1 44.2,52.1
  Bottom 0.406: 39.18,48.99 42.29,52.1 | 42.29,52.1 | 44.2,52.1 SL22.2
  Bottom 0.61: 39.18,48.99 IC8.4
RX-2
  Bottom 0.406: 83.31,63.56 83.41,63.47
  Bottom 0.61: 83.31,63.56 82.58,64.29 70.58,64.29 68.67,62.39 59.53,62.39 58.26,61.12 25.72,61.12 23.65,59.05 19.68,59.05 19.05,58.42 IC2.1 | 83.41,63.47 IC9.2
RXD-1
  Bottom 0.406: 32.86,48.77 32.86,45.91 33.43,45.34 43.15,45.34 44.29,46.48 44.29,47.78 IC8.2
  Bottom 0.61: IC1.1 32.19,55.24 32.86,54.58 32.86,48.77
SCK_IF1
  Bottom 0.406: IC8.26 41.72,41.53 40.2,43.05 18.48,43.05 17.62,42.2 17.62,39.05 16.57,38.01 13.05,38.01 12.48,38.58 10.57,38.58 9.91,37.91 9.91,36.67 10,36.67 11.27,35.4 11.27,34.61 12.38,33.5 16.35,33.5 17.62,32.23 17.62,32.19
  Bottom 0.61: 17.62,32.19 25.92,32.19 R9.1
SCK_IF2  (via drill 0.7)
  Top 0.61: v34.42,33.47 66.42,33.47 67.25,34.29 83.92,34.29 84.49,34.86 84.49,41.15 80.87,44.77 IC9.26
  Bottom 0.61: v34.42,33.47 34.42,33.15 33.66,32.38 29.53,32.38 29.34,32.58 29.34,35.29 C21.2 R27.1
STATUS
  Bottom 0.61: SL22.1 42.26,53.44 IC8.5
TX-2  (via drill 0.7)
  Top 0.61: IC9.3 80.87,52.01 78.87,50.01 52.86,50.01 51.59,51.28 51.59,56.23 49.5,58.33 v48.48,58.33
  Bottom 0.61: IC2.4 26.67,56.99 28.89,59.21 47.62,59.21 48.07,58.77 48.07,58.74 v48.48,58.33
TXD-1
  Bottom 0.406: 35.34,49.05 35.34,46.48 35.81,46.01 41.34,46.01 41.72,46.39 IC8.3
  Bottom 0.61: 35.34,49.05 35.34,51.72 IC1.4
VCC  (via drill 0.7)
  Top 0.61: v42.77,57.05 42.77,56.39 39.4,53.02 v31.43,53.02 | v42.77,57.05 | 72.3,68.1 v72.2,68.2
  Top 0.813: v42.77,65.53 42.77,56.39 | v42.77,65.53 | v72.3,62.01 72.3,68.1
  Bottom 0.61: v42.77,57.05 50.67,57.05 51.15,56.58 R25.1 | 72.26,60.26 72.3,60.29 | R45.2 72.2,70.18 v72.2,68.2 | 31.56,50.4 C5.1 31.43,50.53 | IC5.OUT 68.55,71.99 C4.2 68.81,68.4 C2.+
  Bottom 0.813: IC1.8 32.19,65.53 | v72.3,62.01 72.3,60.29 72.3,57.96 R26.1 70.71,56.37 IC9.7 | 72.26,68.14 v72.2,68.2 72.14,68.14 C2.+ | 72.26,68.14 84.8,68.14 87.6,65.34 JP-7.2 | 72.26,68.14 72.26,68.31 | C18.2 72.26,60.26 | IC2.8 19.05,65.44 19.14,65.53 | IC8.7 31.56,50.4 | v31.43,53.02 31.43,50.53 | v42.77,65.53 46.55,65.53 46.83,65.25 56.67,65.25 57.53,66.1
  Bottom 1.016: C2.+ 66.52,66.1 57.53,66.1 | JP-4.2 10.13,64.52 11.14,65.53 19.14,65.53 32.19,65.53 v42.77,65.53
VDD
  Top 1.016: X1.P$3 19.24,2.25 17.94,0.95 10,0.95 9.53,1.43 9.53,5.4 6.03,8.89 2.38,8.89 0.95,10.32 0.95,27.62 2.06,28.73 3.65,28.73 JP-5.2
  Bottom 1.016: 98.68,28.96 98.68,9.81 97.76,8.89 93.66,8.89 90.96,6.19 90.96,2.54 89.38,0.95 79.85,0.95 | 98.68,28.96 98.68,69.06 97.41,70.33 92.87,70.33 89.44,73.75 X11.P$2 | JP-8.2 96.14,28.96 98.68,28.96 | 79.85,0.95 59.85,0.95 | 59.85,0.95 39.69,0.95 | X2.P$3 39.69,3.75 39.69,0.95 | X3.P$3 59.85,3.78 59.85,0.95 | X4.P$3 79.85,3.87 79.85,0.95 | 39.69,0.95 20.67,0.95 19.24,2.38 X1.P$3
XRES-1
  Bottom 0.61: C6.2 49.7,48.59 | 49.7,48.59 49.21,48.1 47.09,48.1 IC8.1 | R25.2 49.96,48.85 49.7,48.59
XRES-2
  Bottom 0.305: 77.34,61.05 78.96,61.05 79.63,60.39 79.63,59.24 80.3,58.58 81.82,58.58 81.92,58.48
  Bottom 0.406: 82.01,52.2 82.01,54.67 82.55,55.21 82.55,57.78 81.92,58.42 81.92,58.48 | R26.2 75.01,59.82 C17.2 74.98,59.85 76.04,59.85 77.25,61.05 77.34,61.05
  Bottom 0.61: 82.01,52.2 82.77,51.44 84.96,51.44 85.95,52.42 IC9.1

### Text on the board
Top: Top
Bottom: MoBaSbS PM-TDOE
